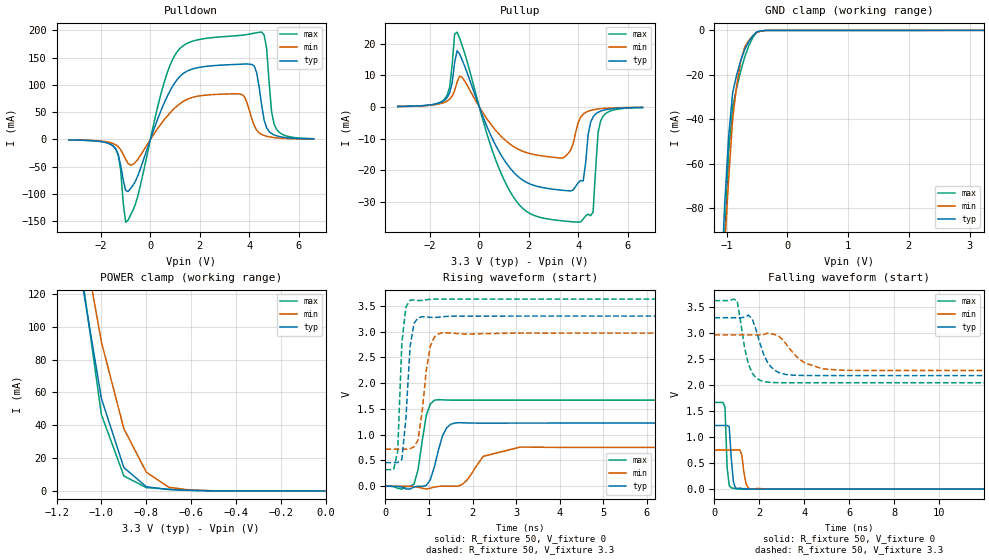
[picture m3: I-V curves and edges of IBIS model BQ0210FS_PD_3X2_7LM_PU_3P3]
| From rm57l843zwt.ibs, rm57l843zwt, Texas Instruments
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|   Model Cell BQ0210FS_PD_3X2_7LM_PU_3P3
|BQ0210FS_PD_3X2_7LM_PU_3P3
[Model]   BQ0210FS_PD_3X2_7LM_PU_3P3
Model_type   I/O
Polarity   Non-Inverting
Enable   Active-Low
Vinl =  1.15
Vinh =  1.55
Cref =  15.0001pF
Rref =  101.0000M
Vref =  0V
Vmeas =  1.65
C_comp   1.2p   1.2p   1.2p
[Model Spec]
Vinl   1.15   1.02   1.28
Vinh   1.55   1.45   1.65
[Temperature Range]   25   155   -40
[Voltage Range]   3.3   2.97   3.63
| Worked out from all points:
|   slope of the pulldown table from 0 to 0.495 V, typ, clamps not added: 8.21 ohm
|   slope of the pullup table from 0 to 0.495 V, typ, clamps not added: 52.1 ohm
|   GND clamp passes 1 mA (typ) near -0.51 V on its own axis
|   POWER clamp passes 1 mA (typ) near -0.71 V on its own axis
|   rising waveform, R_fixture 50, V_fixture 0: 20-80 % time 237ps typ, 451ps min, 180ps max; typ from 0 V to 1.23 V
|   rising waveform, R_fixture 50, V_fixture 3.3: 20-80 % time 134ps typ, 196ps min, 107ps max; typ from 0.458 V to 3.3 V
|   falling waveform, R_fixture 50, V_fixture 0: 20-80 % time 132ps typ, 152ps min, 97.2ps max; typ from 1.23 V to 0 V
|   falling waveform, R_fixture 50, V_fixture 3.3: 20-80 % time 29.5ns typ, 31.8ns min, 18.4ns max; typ from 3.3 V to 0.466 V
[POWER_clamp]
|   voltage   I(typ)   I(min)   I(max)
-3.3V     2.37A      2.626A     3.145A
-1.1V     138.4mA    167.6mA    144.8mA
-1.067V   111mA      142mA      112mA
-1.033V   83.64mA    116.3mA    79.25mA
-1V       56.26mA    90.72mA    46.49mA
-900mV    14.24mA    37.93mA    9.123mA
-800mV    2.552mA    11.42mA    2.024mA
-700mV    820.3uA    2.23mA     1.045mA
-600mV    292.3uA    461.4uA    381uA
-500mV    57.31uA    105uA      65.56uA
0V        413.1pA    9.275nA    341.4pA
[Pulldown]
|   voltage   I(typ)   I(min)   I(max)
-3.3V     -899.6uA   -820.6uA   -837.7uA
-1.4V     -17.27mA   -9.734mA   -17.51mA
-1.2V     -47.62mA   -18.77mA   -56.87mA
-1V       -93.34mA   -36.32mA   -151.7mA
1.1V      110.9mA    62.27mA    162mA
3.6V      138mA      83.62mA    190.9mA
4.1V      137.6mA    38.13mA    194.2mA
4.5V      62.69mA    9.297mA    197.1mA
4.7V      21.72mA    5.946mA    167.7mA
4.9V      10.98mA    4.145mA    51.34mA
5.1V      6.781mA    3.055mA    18.84mA
6.6V      1.042mA    806uA      1.545mA
[Pullup]
|   voltage   I(typ)   I(min)   I(max)
-3.3V     154uA      152.3uA    178.5uA
-1.4V     2.171mA    1.484mA    2.544mA
-900mV    17.81mA    7.857mA    23.72mA
500mV     -9.587mA   -5.844mA   -13.22mA
1.4V      -20.78mA   -12.62mA   -28.76mA
3.4V      -26.42mA   -16.07mA   -36.11mA
4V        -23.95mA   -4.859mA   -36.5mA
4.2V      -23.43mA   -2.288mA   -35.5mA
4.6V      -3.136mA   -899.4uA   -33.27mA
4.8V      -1.694mA   -637.7uA   -8.23mA
5V        -1.071mA   -474.1uA   -2.98mA
6.6V      -155uA     -124.4uA   -196.9uA
[GND_clamp]
|   voltage   I(typ)   I(min)   I(max)
-3.3V     -1.949A    -1.625A    -3.258A
-1.1V     -122.2mA   -133.9mA   -153mA
-1.033V   -79.16mA   -98.31mA   -94.35mA
-966.7mV  -47.75mA   -66.92mA   -54.8mA
-900mV    -27.96mA   -39.72mA   -34.3mA
-833.3mV  -19.96mA   -24.61mA   -25.71mA
-766.7mV  -13.47mA   -13.82mA   -18.2mA
-700mV    -8.48mA    -7.369mA   -11.77mA
-566.7mV  -2.409mA   -2.357mA   -3.204mA
-500mV    -646.1uA   -907.8uA   -753.4uA
-300mV    -20.81uA   -21.53uA   -33.46uA
3.233V    -1.13uA    3.989uA    -9.303uA
[Ramp]
| variable   typ   min   max
dV/dt_f   1.749441/29.49385n   0.5673973/0.3503668n   2.040077/18.38833n
dV/dt_r  0.7842286/0.2504593n  0.4914017/0.410137n   1.054101/0.1905069n
R_load = 50
[Rising Waveform]
R_fixture = 50
V_fixture = 0
V_fixture_min = 0
V_fixture_max = 0
|   time   V(typ)   V(min)   V(max)
0s        118.5uV    107.4uV    121.8uV
656ps     -13.46mV   -7.578mV   40.32mV
748ps     -381uV     -18.14mV   321.8mV
936ps     15.03mV    -53.87mV   1.369V
1.216ns   701.1mV    -2.993mV   1.679V
1.496ns   1.201V     -85.11uV   1.671V
1.872ns   1.228V     118.3mV    1.67V
2.244ns   1.224V     580.4mV    1.67V
3.092ns   1.225V     760.2mV    1.67V
35.52ns   1.225V     753.6mV    1.671V
[Rising Waveform]
R_fixture = 50
V_fixture = 3.3
V_fixture_min = 2.97
V_fixture_max = 3.63
|   time   V(typ)   V(min)   V(max)
0s        457.7mV    717.4mV    321.8mV
188ps     457.5mV    717.5mV    326.8mV
280ps     460.6mV    717.5mV    674.3mV
376ps     523.2mV    716.9mV    2.782V
468ps     1.304V     717.2mV    3.475V
564ps     2.705V     727.9mV    3.607V
748ps     3.267V     897.1mV    3.601V
1.028ns   3.276V     2.712V     3.626V
1.308ns   3.288V     2.974V     3.63V
35.52ns   3.3V       2.97V      3.63V
[Falling Waveform]
R_fixture = 50
V_fixture = 0
V_fixture_min = 0
V_fixture_max = 0
|   time   V(typ)   V(min)   V(max)
0s        1.225V     753.6mV    1.671V
468ps     1.225V     753.6mV    1.58V
564ps     1.226V     753.6mV    413.7mV
656ps     1.205V     753.7mV    69.88mV
844ps     139.6mV    753.9mV    17.75mV
1.028ns   12.73mV    754.3mV    3.074mV
1.216ns   14.03mV    660mV      1.054mV
1.404ns   3.643mV    105.2mV    1.357mV
1.684ns   850.4uV    -26.48uV   1.207mV
35.52ns   286.8uV    259.7uV    136.3uV
[Falling Waveform]
R_fixture = 50
V_fixture = 3.3
V_fixture_min = 2.97
V_fixture_max = 3.63
|   time   V(typ)   V(min)   V(max)
0s        3.3V       2.97V      3.63V
1.008ns   3.299V     2.97V      3.628V
1.512ns   3.35V      2.97V      2.402V
2.18ns    2.606V     2.977V     2.073V
18.06ns   2.186V     2.285V     2.052V
20.81ns   2.186V     2.285V     477.5mV
29.14ns   2.189V     2.285V     345.2mV
34.82ns   551.6mV    2.285V     345mV
35.92ns   525.6mV    755.6mV    345mV
36.8ns    465.6mV    755.6mV    345mV
